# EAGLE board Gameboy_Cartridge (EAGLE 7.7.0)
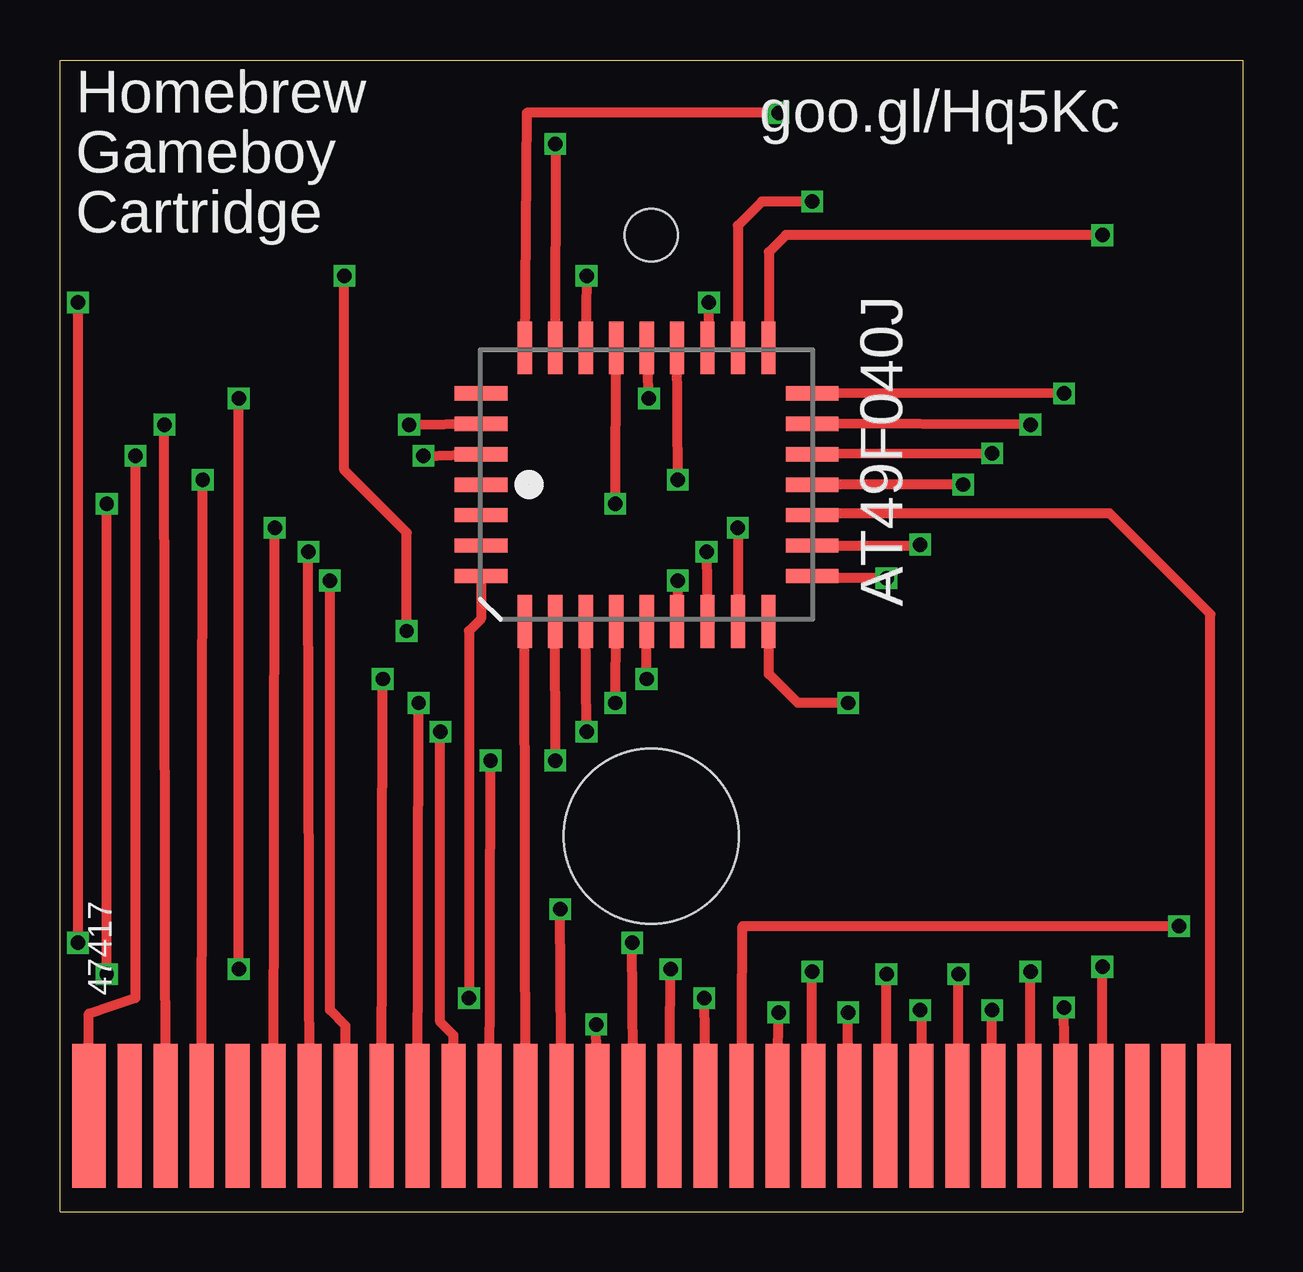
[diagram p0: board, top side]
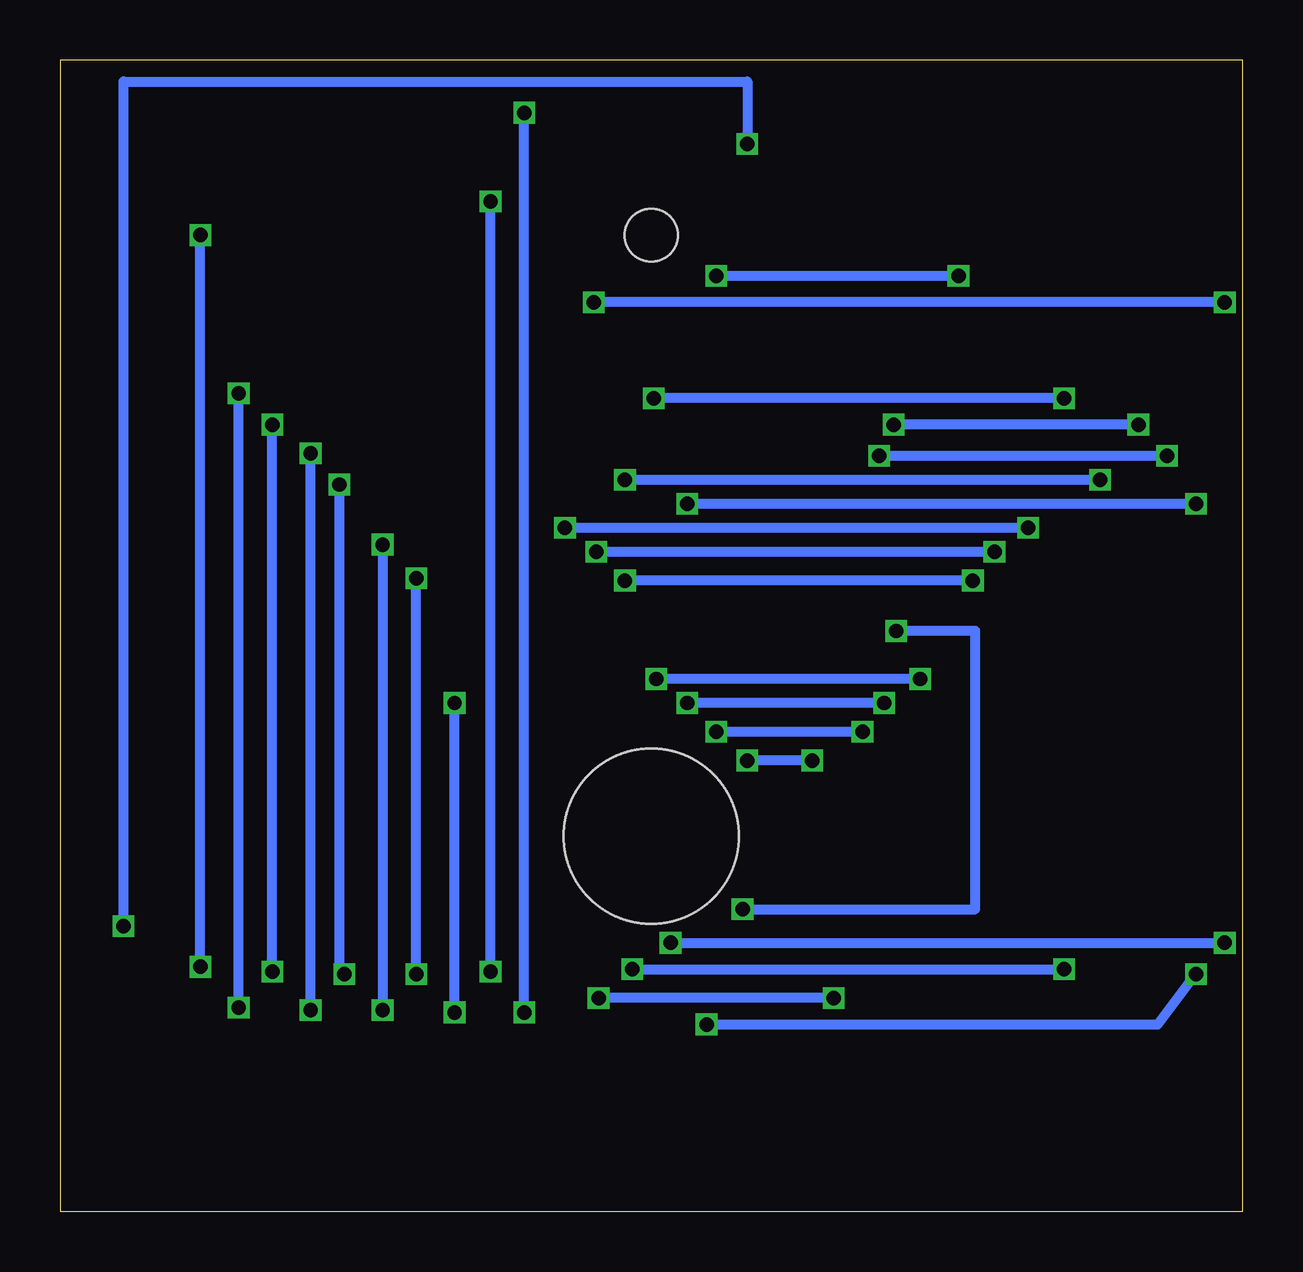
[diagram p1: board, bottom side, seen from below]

Size 49.3 x 48 mm. Coordinates in mm from the lower left corner, seen from the top.
Outline: 49.3,48 49.3,0 0,0 0,48 49.3,48
Copper layers (1*16): Top 0.035mm / dielectric 1.5mm / Bottom 0.035mm
Design rules "SeeedStudio_2layer_DRU_no_angle_20140221": minimum track width 6mil, minimum drill 12mil, track to track 6mil, track to pad 6mil, pad to pad 6mil, via to via 6mil, smd to smd 0mil, copper to edge 10mil, drill to drill 10mil, minimum pad ring 10mil, minimum via ring 6mil, stop-mask expansion 2mil, vias tented up to drill 100mil, thermal gap 10mil
Holes 7.3 mm at 24.65,15.65
Holes 2.2 mm at 24.65,40.7

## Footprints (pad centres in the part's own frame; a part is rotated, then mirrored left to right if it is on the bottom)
PLCC32R = smd 0.6 x 2.2: 1 0,6.9; 2 -1.27,6.9; 3 -2.54,6.9; 4 -3.81,6.9; 14 -3.81,-6.9; 15 -2.54,-6.9; 16 -1.27,-6.9; 17 0,-6.9; 18 1.27,-6.9; 19 2.54,-6.9; 20 3.81,-6.9; 30 3.81,6.9; 31 2.54,6.9; 32 1.27,6.9 | smd 2.2 x 0.6: 5 -5.7,5.08; 6 -5.7,3.81; 7 -5.7,2.54; 8 -5.7,1.27; 9 -5.7,0; 10 -5.7,-1.27; 11 -5.7,-2.54; 12 -5.7,-3.81; 13 -5.7,-5.08; 21 5.7,-5.08; 22 5.7,-3.81; 23 5.7,-2.54; 24 5.7,-1.27; 25 5.7,0; 26 5.7,1.27; 27 5.7,2.54; 28 5.7,3.81; 29 5.7,5.08
CONNECTOR = smd 1.4 x 6: 1 0.7,-3; 32 47.6,-3 | smd 1 x 6: 2 2.4,-3; 3 3.9,-3; 4 5.4,-3; 5 6.9,-3; 6 8.4,-3; 7 9.9,-3; 8 11.4,-3; 9 12.9,-3; 10 14.4,-3; 11 15.9,-3; 12 17.4,-3; 13 18.9,-3; 14 20.4,-3; 15 21.9,-3; 16 23.4,-3; 17 24.9,-3; 18 26.4,-3; 19 27.9,-3; 20 29.4,-3; 21 30.9,-3; 22 32.4,-3; 23 33.9,-3; 24 35.4,-3; 25 36.9,-3; 26 38.4,-3; 27 39.9,-3; 28 41.4,-3; 29 42.9,-3; 30 44.4,-3; 31 45.9,-3

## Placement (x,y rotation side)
IC1  AT49F040J  [PLCC32R]  24.45,30.3 90 top
U$1  CONNECTOR  [CONNECTOR]  0.5,7 0 top

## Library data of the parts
IC1 U$1 = gameboy

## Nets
3: IC1.31 U$1.3
4: IC1.24 U$1.4
5: U$1.5
6: IC1.12 U$1.6
7: IC1.11 U$1.7
8: IC1.10 U$1.8
9: IC1.9 U$1.9
10: IC1.8 U$1.10
11: IC1.7 U$1.11
12: IC1.6 U$1.12
13: IC1.5 U$1.13
14: IC1.27 U$1.14
15: IC1.26 U$1.15
16: IC1.23 U$1.16
17: IC1.25 U$1.17
18: IC1.4 U$1.18
19: IC1.28 U$1.19
20: IC1.29 U$1.20
21: IC1.22 U$1.21
22: IC1.13 U$1.22
23: IC1.14 U$1.23
24: IC1.15 U$1.24
25: IC1.17 U$1.25
26: IC1.18 U$1.26
27: IC1.19 U$1.27
28: IC1.20 U$1.28
29: IC1.21 U$1.29
30: U$1.30
31: U$1.31
GND: IC1.16 U$1.32
VDD: IC1.32 U$1.1

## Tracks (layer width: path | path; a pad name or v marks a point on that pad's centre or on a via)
3  (via drill 0.6)
  Top 0.406: U$1.3 v4.35,32.8 | v14.55,32.8 IC1.31
  Bottom 0.406: v4.35,32.8 v14.55,32.8
4  (via drill 0.6)
  Top 0.406: U$1.4 v5.95,30.5 | v25.75,30.5 IC1.24
  Bottom 0.406: v5.95,30.5 v25.75,30.5
6  (via drill 0.6)
  Top 0.406: U$1.6 v8.95,28.5 | v28.25,28.5 IC1.12
  Bottom 0.406: v8.95,28.5 v28.25,28.5
7  (via drill 0.6)
  Top 0.406: U$1.7 v10.35,27.5 | v26.95,27.5 IC1.11
  Bottom 0.406: v10.35,27.5 v26.95,27.5
8  (via drill 0.6)
  Top 0.406: 11.85,4 U$1.8 11.9,7.75 11.25,8.4 v11.25,26.3 | v25.75,26.3 IC1.10
  Bottom 0.406: v11.25,26.3 v25.75,26.3
9  (via drill 0.6)
  Top 0.406: U$1.9 v13.45,22.2 | v24.45,22.2 IC1.9
  Bottom 0.406: v13.45,22.2 v24.45,22.2
10  (via drill 0.6)
  Top 0.406: U$1.10 v14.95,21.2 | v23.15,21.2 IC1.8
  Bottom 0.406: v14.95,21.2 v23.15,21.2
11  (via drill 0.6)
  Top 0.406: v21.95,20 IC1.7 | U$1.11 16.4,7.35 15.85,7.9 v15.85,20
  Bottom 0.406: v15.85,20 v21.95,20
12  (via drill 0.6)
  Top 0.406: U$1.12 v17.95,18.8 | v20.65,18.8 IC1.6
  Bottom 0.406: v17.95,18.8 v20.65,18.8
13
  Top 0.406: U$1.13 IC1.5
14  (via drill 0.6)
  Top 0.406: v14.45,24.2 14.45,28.3 11.85,30.9 v11.85,39 | v21.95,39 IC1.27 | U$1.14 v20.85,12.6
  Bottom 0.406: v14.45,24.2 11.15,24.2 11.15,12.6 v20.85,12.6 | v11.85,39 v21.95,39
15  (via drill 0.6)
  Top 0.406: U$1.15 v22.35,7.8 | v1.95,9.9 v1.95,29.5 | v23.15,29.5 IC1.26
  Bottom 0.406: v22.35,7.8 3.55,7.8 v1.95,9.9 | v1.95,29.5 v23.15,29.5
16  (via drill 0.6)
  Top 0.406: U$1.16 v23.85,11.2 | v0.75,11.2 v0.75,37.9 | v27.05,37.9 IC1.23
  Bottom 0.406: v23.85,11.2 v0.75,11.2 | v0.75,37.9 v27.05,37.9
17  (via drill 0.6)
  Top 0.406: U$1.17 v25.45,10.1 | v7.45,10.1 v7.45,33.9 | v24.55,33.9 IC1.25
  Bottom 0.406: v25.45,10.1 v7.45,10.1 | v7.45,33.9 v24.55,33.9
18  (via drill 0.6)
  Top 0.406: IC1.4 17.55,24.7 17.05,24.2 v17.05,8.9 | v26.85,8.9 U$1.18
  Bottom 0.406: v17.05,8.9 v26.85,8.9
19  (via drill 0.6)
  Top 0.406: U$1.19 28.45,11.9 v46.65,11.9 | v20.65,44.5 IC1.28
  Bottom 0.406: v46.65,11.9 46.65,47.1 20.65,47.1 v20.65,44.5
20  (via drill 0.6)
  Top 0.406: U$1.20 v29.95,8.3 | v29.95,45.8 19.45,45.8 IC1.29
  Bottom 0.406: v29.95,8.3 v29.95,45.8
21  (via drill 0.6)
  Top 0.406: U$1.21 31.35,4 v31.35,10 | v31.35,42.1 29.25,42.1 28.25,41.1 IC1.22
  Bottom 0.406: v31.35,10 v31.35,42.1
22  (via drill 0.6)
  Top 0.406: U$1.22 32.85,4 v32.85,8.3 | v32.85,21.2 30.75,21.2 29.55,22.4 29.55,24.58 IC1.13
  Bottom 0.406: v32.85,8.3 v32.85,21.2
23  (via drill 0.6)
  Top 0.406: U$1.23 34.45,4 v34.45,9.9 | v34.45,26.4 31.35,26.4 IC1.14
  Bottom 0.406: v34.45,9.9 v34.45,26.4
24  (via drill 0.6)
  Top 0.406: IC1.15 35.85,27.76 v35.85,27.8 | v35.85,8.4 35.9,8.4 U$1.24
  Bottom 0.406: v35.85,27.8 v35.85,8.4
25  (via drill 0.6)
  Top 0.406: U$1.25 37.45,4 v37.45,9.9 | v37.65,30.3 IC1.17
  Bottom 0.406: v37.45,9.9 37.65,9.9 v37.65,30.3
26  (via drill 0.6)
  Top 0.406: U$1.26 38.85,4 v38.85,8.4 | v38.85,31.6 IC1.18
  Bottom 0.406: v38.85,8.4 v38.85,31.6
27  (via drill 0.6)
  Top 0.406: U$1.27 40.45,4 v40.45,10 | v40.45,32.8 IC1.19
  Bottom 0.406: v40.45,10 v40.45,32.8
28  (via drill 0.6)
  Top 0.406: U$1.28 v41.85,8.5 | v41.85,34.1 IC1.20
  Bottom 0.406: v41.85,8.5 v41.85,34.1
29  (via drill 0.6)
  Top 0.406: U$1.29 arc90 43.45,4.05 v43.45,10.2 | v43.45,40.7 30.25,40.7 29.55,40 29.55,36.02 IC1.21
  Bottom 0.406: v43.45,10.2 v43.45,40.7
GND
  Top 0.406: U$1.32 47.95,4 47.95,24.9 43.75,29.1 31.42,29.1 IC1.16
VDD  (via drill 0.6)
  Top 0.406: U$1.1 1.2,8.25 3.15,8.9 v3.15,31.5 | v15.15,31.5 IC1.32
  Bottom 0.406: v3.15,31.5 v15.15,31.5

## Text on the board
tPlace: Homebrew | goo.gl/Hq5Kc | Gameboy | Cartridge | 47417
